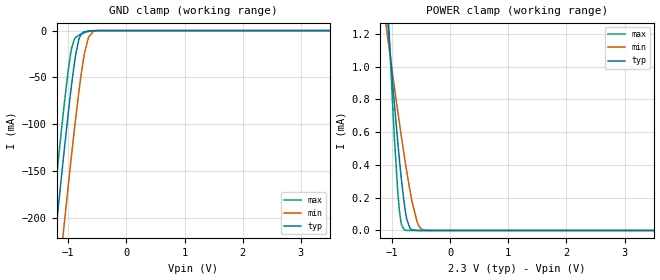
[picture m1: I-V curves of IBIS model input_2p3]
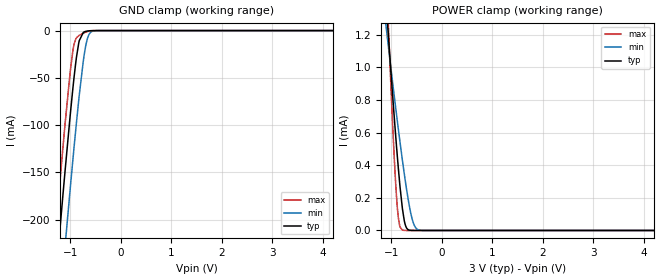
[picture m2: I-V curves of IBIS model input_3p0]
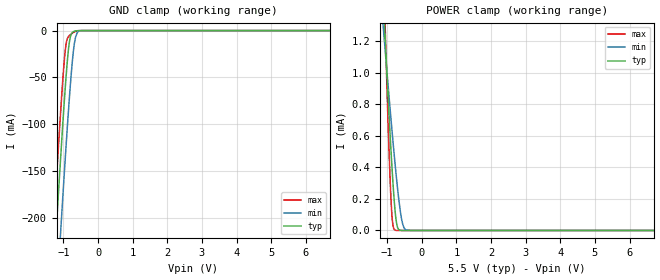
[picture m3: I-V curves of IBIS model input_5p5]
|Texas Instruments Incorporated
| ADS112U04 24-Bit, 4-Channel, 2-kSPS, Delta-Sigma ADC with UART Interface
| Marketing part#   Digital Voltage Range   Package-type   #pins
| ADS112U04RTE   2.3V-5.5V   WQFN   16
| ADS112U04PW   2.3V-5.5V   TSSOP   16
[IBIS Ver]   4.1
[File name]   ads112u04.ibs
[Date]   05/04/2017
[File Rev]   1.0
[Source]
| Texas Instruments Incorporated.
| Analog-eLab Design Center, HPA
| 12500 TI Blvd
| Dallas, TX -75243
[Notes]
| Rev 1.0: 05/04/2017
| - Initial version of the model
| - Model generated from simulations in SPECTRE
| - Model matched to SPICE simulation
| - C_comp although listed in numerical order of value are
|   obtained from varying PVT conditions. For PVT conditions for
|   each specific value refer the buffer description under
|   respective [Model]. IBIS model user is responsible for using
|   appropriate C_comp to simulate for Signal Integrity.
[Disclaimer]
| This model is designed as an aid for customers of Texas Instruments.
| TI and its licensors and suppliers make no warranties, either expressed
| or implied, with respect to this  model, including the warranties of
| merchantability or fitness for a particular purpose. The model is
| provided solely on an "as is" basis. The entire risk as to its quality
| and performance is with the customer.
[Copyright]
(C) Copyright 2017 Texas Instruments Incorporated.All rights reserved.
|   ADS112U04RTE
[Component]   ADS112U04RTE
[Manufacturer]  TI
[Package]   |16 WQFN - RTE package
|   typ   min   max
R_pkg   0   0   0
L_pkg   0   0   0
C_pkg   0   0   0
[Pin]  signal_name model_name   R_pin   L_pin   C_pin
1   RESET   input   NA   NA   NA
2   DGND   gnd   NA   NA   NA
3   AVSS   gnd   NA   NA   NA
4   AIN3   nc   NA   NA   NA
5   AIN2   nc   NA   NA   NA
6   REFN   nc   NA   NA   NA
7   REFP   nc   NA   NA   NA
8   AIN1   nc   NA   NA   NA
9   AIN0   nc   NA   NA   NA
10   AVDD   power   NA   NA   NA
11   DVDD   power   NA   NA   NA
12   GPIO2/DRDY   io   NA   NA   NA
13   TX   output   NA   NA   NA
14   RX   input1   NA   NA   NA
15   GPIO1   io   NA   NA   NA
16   GPIO0   io   NA   NA   NA
|   ADS112U04PW
[Component]   ADS112U04PW
[Manufacturer]  TI
[Package]   |16 TSSOP - PW package
|   typ   min   max
R_pkg   0   0   0
L_pkg   0   0   0
C_pkg   0   0   0
[Pin]  signal_name model_name   R_pin   L_pin   C_pin
1   GPIO1   io   NA   NA   NA
2   GPIO0   io   NA   NA   NA
3   RESET   input   NA   NA   NA
4   DGND   gnd   NA   NA   NA
5   AVSS   gnd   NA   NA   NA
6   AIN3   nc   NA   NA   NA
7   AIN2   nc   NA   NA   NA
8   REFN   nc   NA   NA   NA
9   REFP   nc   NA   NA   NA
10   AIN1   nc   NA   NA   NA
11   AIN0   nc   NA   NA   NA
12   AVDD   power   NA   NA   NA
13   DVDD   power   NA   NA   NA
14   GPIO2/DRDY   io   NA   NA   NA
15   TX   output   NA   NA   NA
16   RX   input1   NA   NA   NA
|   Model Selectors
[Model Selector] input
input_2p3   2.3V   digital Input
input_3p0   3.0V   digital Input
input_5p5   5.5V   digital Input
[Model Selector] input1
input1_2p3   2.3V   digital Input
input1_3p0   3.0V   digital Input
input1_5p5   5.5V   digital Input
[Model Selector] output
output_2p3   2.3V   digital Output
output_3p0   3.0V   digital Output
output_5p5   5.5V   digital Output
[Model Selector] io
io_2p3   2.3V   digital I/O
io_3p0   3.0V   digital I/O
io_5p5   5.5V   digital I/O
| Models and submodels in the file (12): input_2p3 (Input), input_3p0 (Input), input_5p5 (Input), input1_2p3 (Input), input1_3p0 (Input), input1_5p5 (Input), output_2p3 (3-state), output_3p0 (3-state), output_5p5 (3-state), io_2p3 (I/O), io_3p0 (I/O), io_5p5 (I/O)
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|   input_2p3 Model
[Model]   input_2p3
Model_type   Input
Vinl = 0.69
Vinh = 1.61
|   typ   min   max
C_comp   7.30483E-13   6.81776E-13   7.68495E-13
[Model spec]
|subparameter
Vinl   0.69   0.6897   0.6903
Vinh   1.61   1.6093   1.6107
| Where Nom  PVT is Nominal Process, 2.3V, 27C
|   Fast PVT is Strong Process,  2.301V, -40C
|   Slow PVT is Weak Process,   2.299, 125C
[Voltage Range]   2.3   2.299   2.301
[Temperature Range]   27   125   -40
[Power Clamp Reference]   2.3   2.299   2.301
[GND Clamp Reference]   0   0   0
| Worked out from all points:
|   GND clamp passes 1 mA (typ) near -0.70 V on its own axis
|   POWER clamp passes 1 mA (typ) near -1.01 V on its own axis
[GND Clamp]
|   Voltage   I(typ)   I(min)   I(max)
-2.3V     -914.9mA   -992.5mA   -866.7mA
-1.382V   -321.3mA   -401.4mA   -270.9mA
-1.155V   -179.7mA   -259.6mA   -129.5mA
-1.072V   -130.2mA   -209.4mA   -81.15mA
-995.9mV  -86.8mA    -164.3mA   -41.23mA
-940.7mV  -57.44mA   -132.5mA   -19.04mA
-871.7mV  -26.08mA   -94.28mA   -7.305mA
-816.5mV  -9.537mA   -65.77mA   -4.877mA
-740.6mV  -1.91mA    -31.86mA   -2.726mA
-650.9mV  -406.8uA   -7.043mA   -910.5uA
-519.8mV  -22.13uA   -233uA     -44.58uA
4.6V      0A         0A         0A
[POWER Clamp]
|   Voltage   I(typ)   I(min)   I(max)
-2.3V     7.288mA    4.671mA    11.91mA
-1.12V    1.492mA    1.304mA    1.767mA
-1.058V   1.211mA    1.138mA    1.282mA
-1.044V   1.149mA    1.101mA    1.177mA
-961.4mV  790.6uA    884.2uA    590.7uA
-899.3mV  538.9uA    725.9uA    235uA
-844.1mV  335.6uA    589.4uA    49.41uA
-788.9mV  165uA      458.3uA    4.283uA
-692.3mV  14.42uA    248.4uA    31.31nA
-568.1mV  131.3nA    53.88uA    0A
-450.8mV  0A         3.106uA    0A
4.6V      0A         0A         0A
|   input_3p0 Model
[Model]   input_3p0
Model_type   Input
Vinl = 0.9
Vinh = 2.1
|   typ   min   max
C_comp   7.07349E-13   6.57113E-13   7.47558E-13
[Model spec]
|subparameter
Vinl   0.9   0.8997   0.9003
Vinh   2.1   2.0993   2.1007
| Where Nom  PVT is Nominal Process, 3.0V, 27C
|   Fast PVT is Strong Process,  3.001V, -40C
|   Slow PVT is Weak Process,   2.999, 125C
[Voltage Range]   3   2.999   3.001
[Temperature Range]   27   125   -40
[Power Clamp Reference]   3   2.999   3.001
[GND Clamp Reference]   0   0   0
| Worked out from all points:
|   GND clamp passes 1 mA (typ) near -0.70 V on its own axis
|   POWER clamp passes 1 mA (typ) near -1.01 V on its own axis
[GND Clamp]
|   Voltage   I(typ)   I(min)   I(max)
-3V       -1.375A    -1.45A     -1.328A
-1.317V   -280.2mA   -360.4mA   -229.6mA
-1.155V   -179.9mA   -259.9mA   -129.7mA
-1.101V   -147.5mA   -227mA     -97.84mA
-1.002V   -90.18mA   -167.9mA   -44.16mA
-930mV    -52.09mA   -126.4mA   -15.99mA
-876mV    -27.77mA   -96.59mA   -7.609mA
-831mV    -12.88mA   -73.02mA   -5.371mA
-723mV    -1.396mA   -25.38mA   -2.299mA
-633mV    -290.5uA   -4.673mA   -671.7uA
-498mV    -12.62uA   -127.9uA   -23.31uA
6V        0A         0A         0A
[POWER Clamp]
|   Voltage   I(typ)   I(min)   I(max)
-3V       10.82mA    6.729mA    18.02mA
-1.101V   1.406mA    1.253mA    1.617mA
-1.065V   1.243mA    1.157mA    1.336mA
-1.02V    1.043mA    1.037mA    998.2uA
-939mV    698.1uA    826.9uA    450.8uA
-885mV    484.3uA    690.5uA    172.1uA
-831mV    291.7uA    558.1uA    29.42uA
-777mV    134.9uA    431.2uA    2.404uA
-705mV    22.06uA    274.3uA    61.99nA
-588mV    287.5nA    75.89uA    0A
-435mV    0A         1.989uA    0A
6V        0A         0A         0A
|   input_5p5 Model
[Model]   input_5p5
Model_type   Input
Vinl = 1.65
Vinh = 3.85
|   typ   min   max
C_comp   6.54074E-13   6.02058E-13   6.91253E-13
[Model spec]
|subparameter
Vinl   1.65   1.6497   1.6503
Vinh   3.85   3.8493   3.8507
| Where Nom  PVT is Nominal Process, 5.5V, 27C
|   Fast PVT is Strong Process,  5.501V, -40C
|   Slow PVT is Weak Process,   5.499, 125C
[Voltage Range]   5.5   5.499   5.501
[Temperature Range]   27   125   -40
[Power Clamp Reference]   5.5   5.499   5.501
[GND Clamp Reference]   0   0   0
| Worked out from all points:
|   GND clamp passes 1 mA (typ) near -0.70 V on its own axis
|   POWER clamp passes 1 mA (typ) near -1.01 V on its own axis
[GND Clamp]
|   Voltage   I(typ)   I(min)   I(max)
-5.5V     -3.028A    -3.1A      -2.983A
-1.375V   -316.7mA   -396.8mA   -266.2mA
-1.243V   -234mA     -314.2mA   -183.5mA
-1.194V   -203.5mA   -283.5mA   -153mA
-1.111V   -153.4mA   -233mA     -103.7mA
-1.045V   -114.6mA   -193.3mA   -66.35mA
-946mV    -60.14mA   -135.5mA   -20.73mA
-830.5mV  -12.75mA   -72.77mA   -5.353mA
-682mV    -700.8uA   -13.19mA   -1.431mA
-599.5mV  -146.1uA   -2.018mA   -345.4uA
-451mV    -3.532uA   -35uA      -5.166uA
11V       0A         0A         0A
[POWER Clamp]
|   Voltage   I(typ)   I(min)   I(max)
-5.5V     23.46mA    14.23mA    39.8mA
-1.111V   1.453mA    1.282mA    1.698mA
-1.045V   1.155mA    1.105mA    1.186mA
-946mV    728.4uA    846.2uA    495uA
-880mV    466.7uA    679.2uA    152.9uA
-830.5mV  291uA      558uA      28.98uA
-764.5mV  106.7uA    403.8uA    1.302uA
-698.5mV  17.92uA    261.9uA    38.57nA
-599.5mV  449nA      90.94uA    0A
-517mV    8.012nA    18.19uA    0A
-451mV    0A         3.146uA    0A
11V       0A         0A         0A
